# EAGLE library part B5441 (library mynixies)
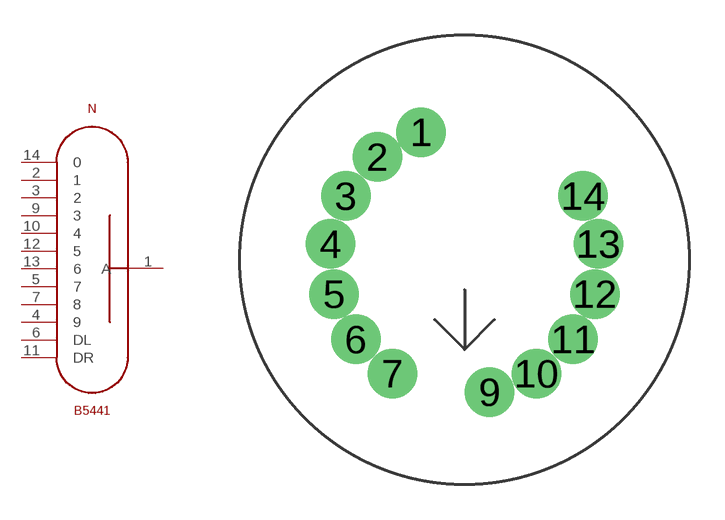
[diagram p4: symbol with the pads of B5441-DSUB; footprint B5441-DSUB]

Designator prefix N

## B5441  [B5441-DSUB]
1  A  pas
2  1  pas
3  2  pas
4  9  pas
5  7  pas
6  DL  pas
7  8  pas
9  3  pas
10  4  pas
11  DR  pas
12  5  pas
13  6  pas
14  0  pas

## Footprint B5441-DSUB (pad centres in mm)
drill 1.4 pad 1.8: 1 -1.837,5.412; 2 -3.693,4.362; 3 -5.034,2.705; 4 -5.675,0.672; 5 -5.527,-1.455; 6 -4.609,-3.379; 7 -3.05,-4.833; 9 1.066,-5.615; 10 3.05,-4.833; 11 4.609,-3.379; 12 5.527,-1.455; 13 5.675,0.672; 14 5.034,2.705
